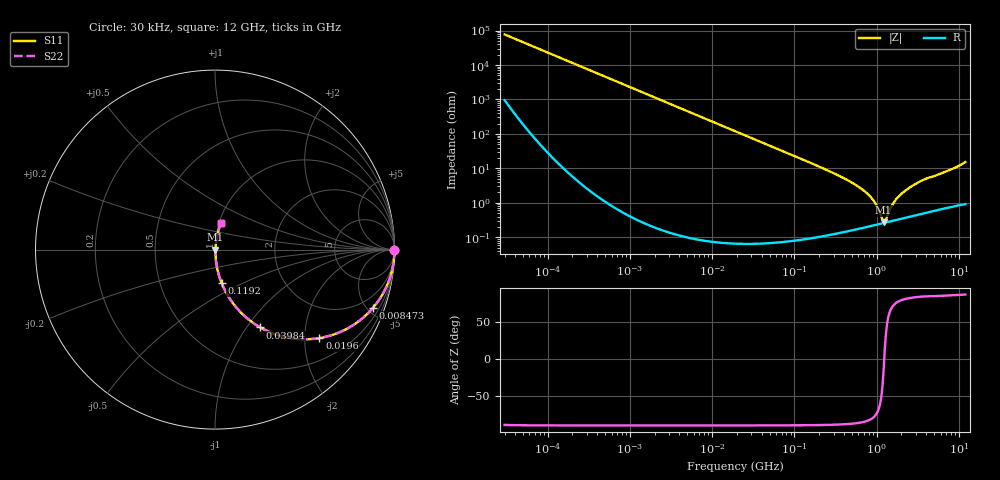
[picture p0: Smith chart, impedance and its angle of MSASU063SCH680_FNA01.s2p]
! MSASU063SCH680_FNA01  S-PARAMETER MODEL  ( General Type )
! Model Generated by TAIYO YUDEN Corporation (http://www.ty-top.com)
! Version 4.0
! TAIYO YUDEN Control No. 120810
! Copyright(c) 2002 TAIYO YUDEN CO.,LTD. All Rights Reserved.
! Product Description (link to TY-COMPAS)
! https://ds.yuden.co.jp/TYCOMPAS/or/detail?pn=MSASU063SCH680JFNA01&u=M
! Products Name : Multilayer Ceramic Capacitors
! Characteristics :
!  Capacitance : 68 pF , Rated Voltage : 50V , TCC : CH / C0H
!  Case Size : 0.6 x 0.3 / 0.024 x 0.012 [mm/inch] , Thickness : 0.3 / 0.012 [mm/inch]
!  (Conditions: Temperature = 25 degC , DC Bias Current/Voltage = 0A / 0V)
! External Node Assignments :
!  1  o---| |---o  2
! GND o---------o GND
! Frequency Range : 0.03MHz  -  12000MHz  [ 401 STEP ]
# MHz S RI R 50
! Freq[MHz].  S11 Real  S11 Imag  S21 Real  S21 Imag  S12 Real  S12 Imag  S22 Real  S22 Imag
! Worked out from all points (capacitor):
!   401 points, 30 kHz to 12 GHz, reference 50 ohm
!   read as one part in series: C = 68.9 pF near 32 kHz
!   lowest |Z| = 270 mohm at 1.216 GHz (marker M1)
!   series resonance near 1.238 GHz, so ESL is about 240 pH
!   S11 on the Smith chart (normalised r, x): 30 kHz: open; 8.473 MHz: 1.00, -5.46; 19.6 MHz: 1.00, -2.36; 39.84 MHz: 1.00, -1.16; 119.2 MHz: 1.00, -0.38; 12 GHz: 1.02, +0.30
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0.03  1 -0.0013  1.77e-05 0.0013  1.77e-05 0.0013  1 -0.0013
0.260295  0.9999 -0.0113  0.000131 0.0113  0.000131 0.0113  0.9999 -0.0113
2.258455  0.9905 -0.0968  0.00947 0.0968  0.00947 0.0968  0.9905 -0.0968
4.897055  0.957 -0.2028  0.043 0.2028  0.043 0.2028  0.957 -0.2028
8.472713  0.8814 -0.3231  0.1186 0.3231  0.1186 0.3231  0.8814 -0.3231
18.97367  0.5972 -0.4902  0.4028 0.4902  0.4028 0.4902  0.5972 -0.4902
19.5955  0.5816 -0.493  0.4184 0.493  0.4184 0.493  0.5816 -0.493
39.83545  0.2517 -0.4334  0.7483 0.4334  0.7483 0.4334  0.2517 -0.4334
64.61702  0.1134 -0.316  0.8866 0.316  0.8866 0.316  0.1134 -0.316
119.2463  0.0363 -0.1849  0.9637 0.1849  0.9637 0.1849  0.0363 -0.1849
164.6252  0.0196 -0.1351  0.9804 0.1351  0.9804 0.1351  0.0196 -0.1351
406.107  0.00399 -0.0505  0.996 0.0505  0.996 0.0505  0.00399 -0.0505
680.3351  0.00243 -0.0237  0.9976 0.0237  0.9976 0.0237  0.00243 -0.0237
939.2353  0.00234 -0.0105  0.9977 0.0105  0.9977 0.0105  0.00234 -0.0105
1215.67  0.00259 -0.000752  0.9974 0.000752  0.9974 0.000752  0.00259 -0.000752
1296.659  0.00269 0.00173  0.9973 -0.00173  0.9973 -0.00173  0.00269 0.00173
1428.372  0.00287 0.00523  0.9971 -0.00523  0.9971 -0.00523  0.00287 0.00523
1625.032  0.00316 0.00972  0.9968 -0.00972  0.9968 -0.00972  0.00316 0.00972
1848.769  0.00351 0.0146  0.9965 -0.0146  0.9965 -0.0146  0.00351 0.0146
2635.962  0.00491 0.0292  0.9951 -0.0292  0.9951 -0.0292  0.00491 0.0292
3758.338  0.00714 0.0465  0.9929 -0.0465  0.9929 -0.0465  0.00714 0.0465
12000  0.0312 0.1461  0.9688 -0.1461  0.9688 -0.1461  0.0312 0.1461
